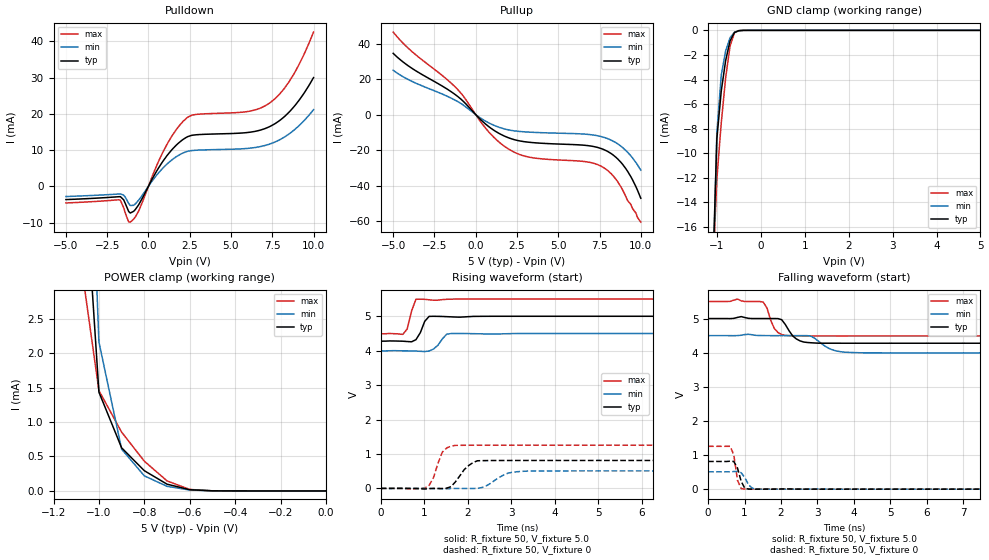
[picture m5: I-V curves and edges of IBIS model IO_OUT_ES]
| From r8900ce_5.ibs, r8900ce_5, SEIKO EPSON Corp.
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[Model]   IO_OUT_ES
Model_type 3-state
Enable Active-High
Polarity Non-Inverting
Vmeas=2.50
C_comp   2.5p   2p   3p
[Temperature Range] 25   85   -40
[Voltage Range]   5.0   4.5   5.5
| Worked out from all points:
|   slope of the pulldown table from 0 to 0.75 V, typ, clamps not added: 124 ohm
|   slope of the pullup table from 0 to 0.75 V, typ, clamps not added: 116 ohm
|   GND clamp passes 1 mA (typ) near -0.71 V on its own axis
|   POWER clamp passes 1 mA (typ) near -0.95 V on its own axis
|   falling waveform, R_fixture 50, V_fixture 5.0: 20-80 % time 303ps typ, 433ps min, 212ps max; typ from 5 V to 4.28 V
|   falling waveform, R_fixture 50, V_fixture 0: 20-80 % time 150ps typ, 179ps min, 105ps max; typ from 0.812 V to 0 V
|   rising waveform, R_fixture 50, V_fixture 5.0: 20-80 % time 153ps typ, 201ps min, 131ps max; typ from 4.28 V to 5 V
|   rising waveform, R_fixture 50, V_fixture 0: 20-80 % time 312ps typ, 397ps min, 216ps max; typ from 0 V to 0.812 V
[Pullup]
-5V       34.51mA    24.97mA    46.48mA
-3.9V     26.29mA    18.87mA    35.82mA
-1.1V     10.27mA    7.384mA    14.21mA
600mV     -5.354mA   -3.707mA   -7.68mA
1.7V      -11.94mA   -7.963mA   -17.58mA
3.2V      -15.54mA   -9.848mA   -23.91mA
6.7V      -17.37mA   -11.07mA   -26.58mA
7.7V      -19.47mA   -12.63mA   -29.58mA
8.3V      -22.58mA   -14.82mA   -34.21mA
8.9V      -28.03mA   -18.56mA   -42.46mA
9.5V      -36.73mA   -24.41mA   -52.95mA
10V       -47.13mA   -31.3mA    -60.6mA
[Pulldown]
-5V       -3.662mA   -2.821mA   -4.594mA
-1.7V     -2.853mA   -2.102mA   -3.849mA
-1.2V     -6.922mA   -4.703mA   -9.822mA
-1.1V     -7.372mA   -5.283mA   -9.897mA
-600mV    -5.148mA   -3.864mA   -6.884mA
900mV     7.06mA     5.145mA    9.637mA
2.1V      12.93mA    9.207mA    17.92mA
2.7V      14.11mA    9.891mA    19.68mA
5.9V      14.79mA    10.41mA    20.55mA
7.3V      16.37mA    11.58mA    22.84mA
8.6V      20.84mA    14.72mA    29.41mA
10V       29.98mA    21.13mA    42.53mA
[GND Clamp]
-5V       -845.9mA   -709.5mA   -1.06A
-1.1V     -20.64mA   -22.12mA   -20.39mA
-1V       -8.831mA   -8.329mA   -12.11mA
-900mV    -4.941mA   -3.657mA   -7.543mA
-800mV    -2.459mA   -1.675mA   -3.865mA
-700mV    -864uA     -604.2uA   -1.29mA
-600mV    -179.5uA   -151uA     -195.7uA
-500mV    -26.95uA   -29.51uA   -18.23uA
-400mV    -3.685uA   -4.954uA   -1.653uA
5V        263.5pA    1.889uA    79.69pA
[POWER Clamp]
-5V       662.7mA    555.2mA    838.5mA
-1.1V     6.482mA    10.72mA    3.807mA
-1V       1.434mA    2.163mA    1.457mA
-900mV    625.6uA    606.7uA    853.6uA
-800mV    293.7uA    218.9uA    432uA
-700mV    98.19uA    66.89uA    145.6uA
-600mV    17.36uA    13.33uA    21.68uA
-500mV    1.719uA    1.889uA    1.298uA
0V        263.5pA    827.2pA    98.57pA
[Falling Waveform]
R_fixture=50
V_fixture=5.0
V_fixture_min=4.5
V_fixture_max=5.5
0s        5V         4.5V       5.5V
1.515ns   5V         4.501V     5.481V
1.616ns   5V         4.5V       5.311V
1.818ns   5V         4.5V       4.71V
2.121ns   4.824V     4.5V       4.507V
2.424ns   4.402V     4.5V       4.494V
2.828ns   4.29V      4.48V      4.491V
3.333ns   4.277V     4.117V     4.492V
3.737ns   4.277V     4.016V     4.491V
10ns      4.277V     3.994V     4.492V
[Falling Waveform]
R_fixture=50
V_fixture=0
V_fixture_min=0
V_fixture_max=0
0s        811.9mV    509.2mV    1.256V
606.1ps   819.7mV    508.4mV    1.256V
707.1ps   811mV      516.6mV    1.004V
808.1ps   618.3mV    521.5mV    259.3mV
909.1ps   227.8mV    480.2mV    18.5mV
1.01ns    23.79mV    334.9mV    405.5uV
1.111ns   4.186mV    128.3mV    35.8uV
1.212ns   454.7uV    30mV       16.5uV
1.313ns   110uV      857.3uV    111.3uV
10ns      -9.834uV   4.787uV    -17.24uV
[Rising Waveform]
R_fixture=50
V_fixture=5.0
V_fixture_min=4.5
V_fixture_max=5.5
0s        4.277V     3.994V     4.492V
505.1ps   4.276V     3.996V     4.473V
606.1ps   4.266V     3.995V     4.628V
707.1ps   4.258V     3.994V     5.152V
808.1ps   4.32V      3.989V     5.495V
1.01ns    4.854V     3.977V     5.493V
1.111ns   4.997V     3.99V      5.478V
1.515ns   4.989V     4.48V      5.493V
1.616ns   4.983V     4.499V     5.497V
10ns      5V         4.5V       5.5V
[Rising Waveform]
R_fixture=50
V_fixture=0
V_fixture_min=0
V_fixture_max=0
0s        0V         0V         0V
1.01ns    -17.96mV   97.46uV    10.82mV
1.212ns   -989.6uV   -3.013mV   314.1mV
1.414ns   -2.157mV   -11.82mV   1.051V
1.717ns   192.5mV    -228.4uV   1.25V
1.919ns   547.7mV    -1.227mV   1.253V
2.222ns   802.5mV    878.2uV    1.255V
2.929ns   811.1mV    444.8mV    1.256V
3.333ns   811.8mV    500.6mV    1.256V
10ns      811.9mV    509.2mV    1.256V
[Ramp]
R_load=50
dV/dt_r   4.872E-1/3.048E-10   3.055E-1/3.899E-10   7.534E-1/1.988E-10
dV/dt_f   4.338E-1/2.920E-10   3.035E-1/4.276E-10   6.051E-1/2.108E-10
|[End   IO_OUT_ES
